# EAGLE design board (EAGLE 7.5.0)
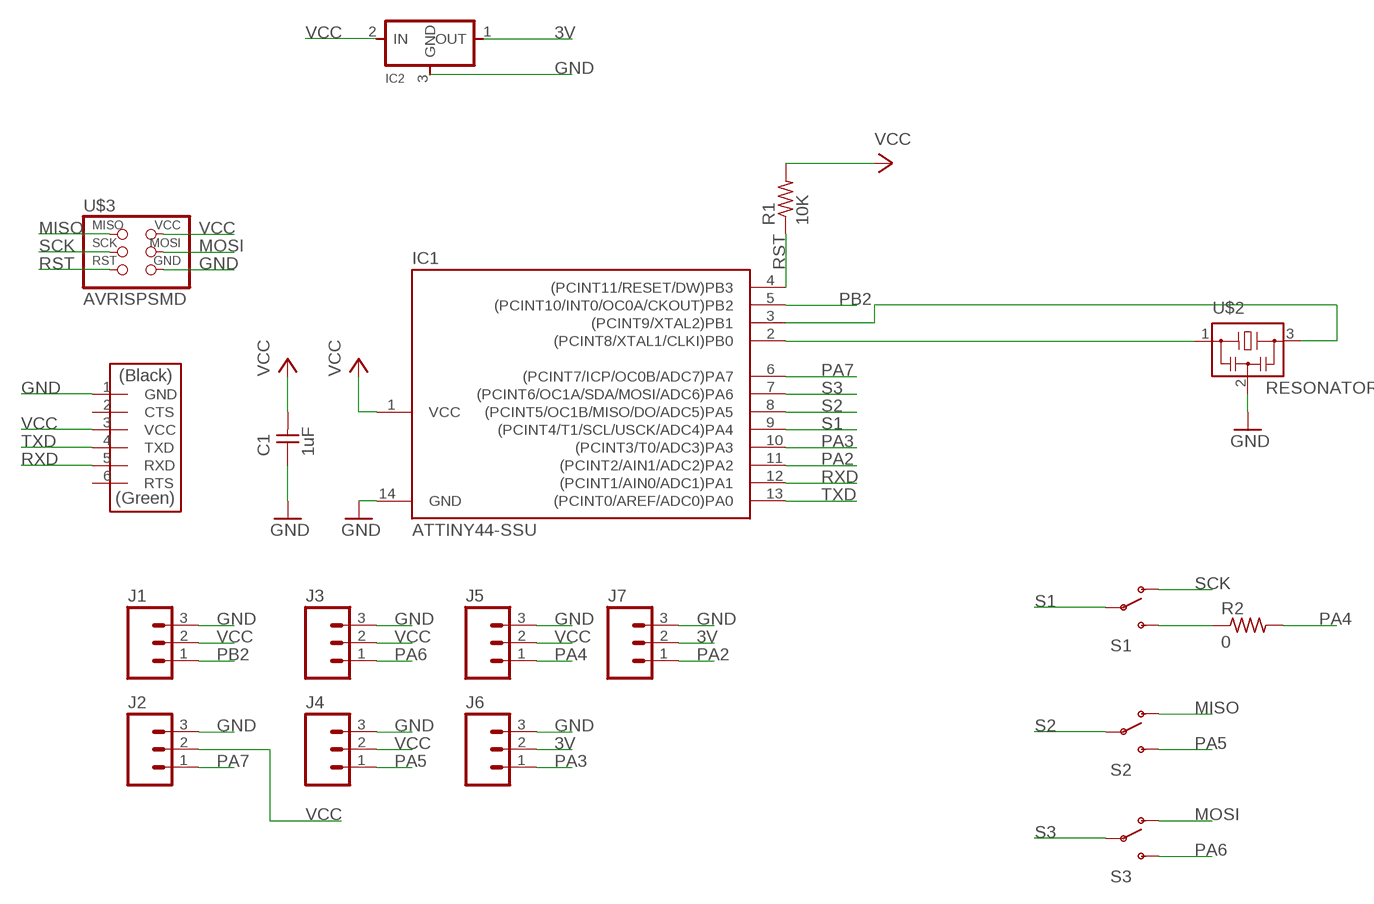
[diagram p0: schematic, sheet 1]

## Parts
C1  1uF  CAP-UNPOLARIZED  [C1206]
IC1  ATTINY44-SSU  [SOIC14]
IC2  REGULATORSOT23  [SOT23]
J1  M03SMD_RA_MALE  [1X03_SMD_RA_MALE]
J2  M03SMD_RA_MALE  [1X03_SMD_RA_MALE]
J3  M03SMD_RA_MALE  [1X03_SMD_RA_MALE]
J4  M03SMD_RA_MALE  [1X03_SMD_RA_MALE]
J5  M03SMD_RA_MALE  [1X03_SMD_RA_MALE]
J6  M03SMD_RA_MALE  [1X03_SMD_RA_MALE]
J7  M03SMD_RA_MALE  [1X03_SMD_RA_MALE]
R1  10K  RES-US1206FAB  [R1206FAB]
R2  0  RES-US1206FAB  [R1206FAB]
S1  SWITCH-SPDTSMD2  [SWITCH-SPDT-SMD]
S2  SWITCH-SPDTSMD2  [SWITCH-SPDT-SMD]
S3  SWITCH-SPDTSMD2  [SWITCH-SPDT-SMD]
U$2  RESONATOR  [EFOBM]
U$3  AVRISPSMD  [2X03SMD]
U$4  FTDI-SMD-HEADER  [1X06SMD]

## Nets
3V: IC2.1(OUT) J6.2 J7.2
GND: C1.1 IC1.14(GND) IC2.3(GND) J1.3 J2.3 J3.3 J4.3 J5.3 J6.3 J7.3 U$2.2 U$3.6(GND) U$4.1(GND)
MISO: S2.1(O) U$3.1(MISO)
MOSI: S3.1(O) U$3.4(MOSI)
N$1: IC1.3((PCINT9/XTAL2)PB1) U$2.3
N$2: IC1.2((PCINT8/XTAL1/CLKI)PB0) U$2.1
N$3: R2.1 S1.3(S)
PA2: IC1.11((PCINT2/AIN1/ADC2)PA2) J7.1
PA3: IC1.10((PCINT3/T0/ADC3)PA3) J6.1
PA4: J5.1 R2.2
PA5: J4.1 S2.3(S)
PA6: J3.1 S3.3(S)
PA7: IC1.6((PCINT7/ICP/OC0B/ADC7)PA7) J2.1
PB2: IC1.5((PCINT10/INT0/OC0A/CKOUT)PB2) J1.1
RST: IC1.4((PCINT11/RESET/DW)PB3) R1.1 U$3.5(RST)
RXD: IC1.12((PCINT1/AIN0/ADC1)PA1) U$4.5(RXD)
S1: IC1.9((PCINT4/T1/SCL/USCK/ADC4)PA4) S1.2(P)
S2: IC1.8((PCINT5/OC1B/MISO/DO/ADC5)PA5) S2.2(P)
S3: IC1.7((PCINT6/OC1A/SDA/MOSI/ADC6)PA6) S3.2(P)
SCK: S1.1(O) U$3.3(SCK)
TXD: IC1.13((PCINT0/AREF/ADC0)PA0) U$4.4(TXD)
VCC: C1.2 IC1.1(VCC) IC2.2(IN) J1.2 J2.2 J3.2 J4.2 J5.2 R1.2 U$3.2(VCC) U$4.3(VCC)
Unconnected: U$4.2(CTS) U$4.6(RTS)

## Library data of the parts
C1 = fab:CAP-UNPOLARIZED
IC1 = fab:ATTINY44
IC2 = fab:REGULATOR
J1-J7 = SparkFun-Connectors:M03: Header 3 Standard 3-pin 0.1" header. Use with straight break away headers (SKU : PRT-00116), right angle break away headers (PRT-00553), swiss pins (PRT-00743), machine pins (PRT-00117), and female headers (PRT-00115). Molex polarized connector foot print use with SKU : PRT-08232 with associated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; PROD_ID: CONN-10925
R1 R2 = fab:RES-US: Resistor (US Symbol)
S1-S3 = SparkFun-Electromechanical:SWITCH-SPDT: SPDT Switch Simple slide switch, Spark Fun Electronics SKU : COM-00102 DPDT SMT slide switch, AYZ0202, SWCH-08179
U$2 = fab:RESONATOR
U$3 = fab:AVRISP
U$4 = fab:FTDI-SMD-HEADER

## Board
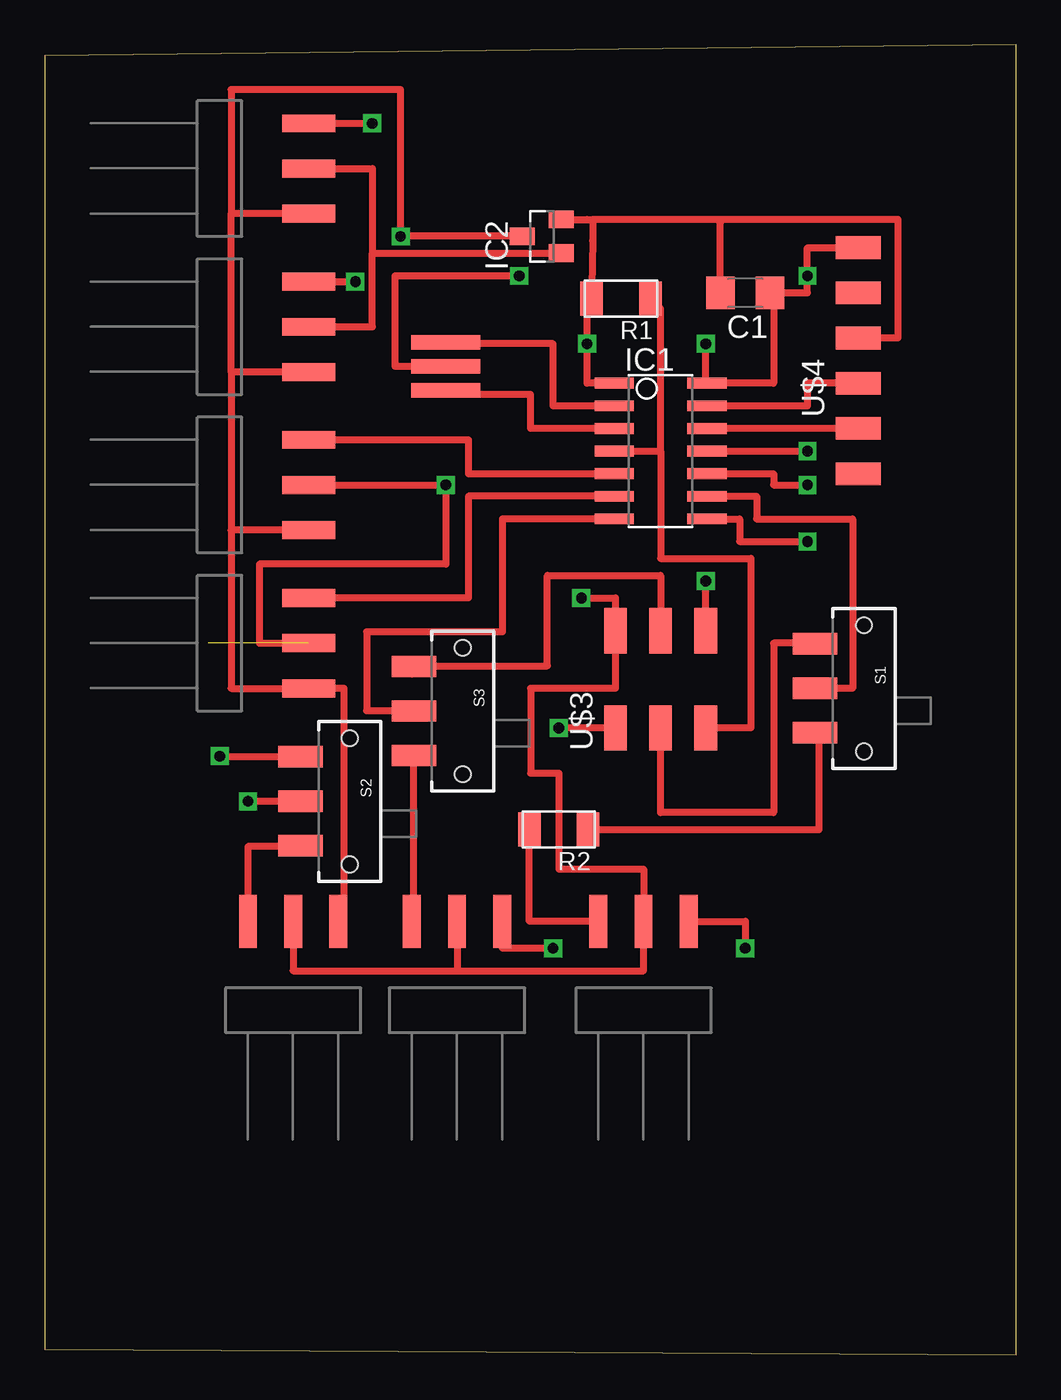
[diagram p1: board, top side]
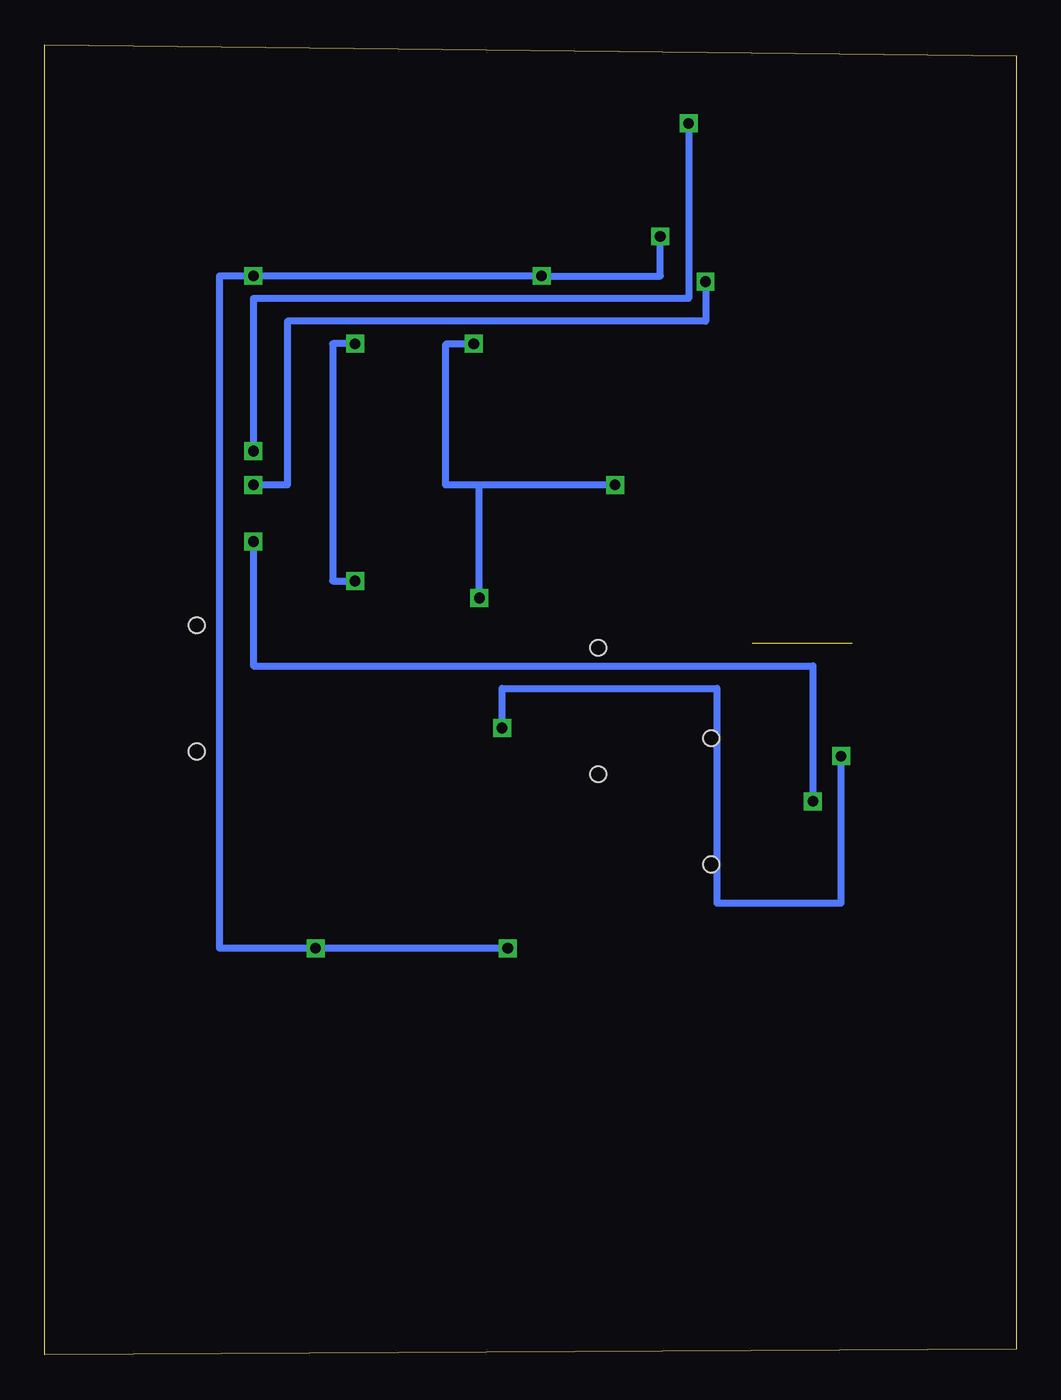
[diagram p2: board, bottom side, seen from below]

Size 54.6 x 73.65 mm. Coordinates in mm from the lower left corner, seen from the top.
Outline: 0,0.32 54.6,0 54.6,73.65 0,73.02 0,0.32
Copper layers (1*16): Top 0.035mm / dielectric 1.5mm / Bottom 0.035mm
Design rules "default": minimum track width 10mil, minimum drill 24mil, track to track 8mil, track to pad 8mil, pad to pad 8mil, via to via 8mil, smd to smd 8mil, copper to edge 40mil, drill to drill 8mil, minimum pad ring 10mil, minimum via ring 8mil, stop-mask expansion 4mil, vias tented up to drill 0mil, thermal gap 10mil

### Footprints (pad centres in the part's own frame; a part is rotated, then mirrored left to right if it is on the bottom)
C1206 = smd 1.6 x 1.8: 1 -1.4,0; 2 1.4,0
SOIC14 = smd 0.61 x 2.21: 1 -3.81,-2.603; 2 -2.54,-2.603; 3 -1.27,-2.603; 4 0,-2.603; 5 1.27,-2.603; 6 2.54,-2.603; 7 3.81,-2.603; 8 3.81,2.603; 9 2.54,2.603; 10 1.27,2.603; 11 0,2.603; 12 -1.27,2.603; 13 -2.54,2.603; 14 -3.81,2.603
SOT23 = smd 1 x 1.4: 1 -0.95,-1.1; 2 0.95,-1.1; 3 0,1.1
1X03_SMD_RA_MALE = smd 1 x 3: 1 -2.54,5; 2 0,5; 3 2.54,5
R1206FAB = smd 1.27 x 1.905: 1 -1.651,0; 2 1.651,0
SWITCH-SPDT-SMD = smd 1.2 x 2.5: 1 -2.5,-2.75; 2 0,-2.75; 3 2.5,-2.75 | hole 0.9: -3.55,0; 3.55,0
EFOBM = smd 0.8 x 3.9: 1 -1.35,0; 2 0,0; 3 1.35,0
2X03SMD = smd 2.54 x 1.27: 1 -2.54,2.54; 2 2.92,2.54; 3 -2.54,0; 4 2.92,0; 5 -2.54,-2.54; 6 2.92,-2.54
1X06SMD = smd 2.54 x 1.27: 1 0,6.35; 2 0,3.81; 3 0,1.27; 4 0,-1.27; 5 0,-3.81; 6 0,-6.35

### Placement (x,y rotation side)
C1  39.37,59.69 180 top
IC1  34.61,50.8 270 top
IC2  27.94,62.87 90 top
J1  9.84,48.9 270 top
J2  9.84,40.01 270 top
J3  23.18,19.37 0 top
J4  13.97,19.37 0 top
J5  33.66,19.37 0 top
J6  9.84,57.79 270 top
J7  9.84,66.67 270 top
R1  32.38,59.37 180 top
R2  28.89,29.53 180 top
S1  46.04,37.47 270 top
S2  17.14,31.11 270 top
S3  23.5,36.2 270 top
U$2  22.54,55.56 270 top
U$3  34.61,37.78 90 top
U$4  45.72,55.88 0 top

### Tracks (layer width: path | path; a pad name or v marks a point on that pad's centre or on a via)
3V
  Top 0.406: 18.41,61.91 25.23,61.91 IC2.1 | J6.2 18.41,57.79 18.41,61.91 | J7.2 18.41,66.68 18.41,61.91
GND  (via drill 0.6)
  Top 0.406: IC2.3 v20,62.86 20,71.12 10.48,71.12 10.48,64.14 | v37.15,56.83 37.15,54.61 IC1.14 40.96,54.61 40.96,59.69 C1.1 42.86,59.69 v42.86,60.64 42.86,62.23 U$4.1 | U$3.6 v37.15,43.5 | J6.3 10.48,55.25 | 10.48,55.25 10.48,64.14 | J7.3 10.48,64.14 | 10.48,55.25 10.48,46.36 | J1.3 10.48,46.36 | 10.48,46.36 10.48,37.47 J2.3 16.83,37.47 16.83,24.68 J4.3 | J5.3 39.37,24.37 v39.37,22.86 | v28.57,22.86 25.72,22.86 J3.3 | v26.67,60.64 19.68,60.64 19.68,55.56 U$2.2
  Bottom 0.406: v37.15,56.83 38.42,56.83 38.42,43.5 v37.15,43.5 | v28.57,22.86 v39.37,22.86 44.77,22.86 44.77,60.64 v42.86,60.64 v26.67,60.64 20,60.64 v20,62.86
MISO  (via drill 0.6)
  Top 0.406: U$3.1 v28.89,35.24 | S2.1 10.16,33.61 v9.84,33.65
  Bottom 0.406: v28.89,35.24 28.89,37.47 16.83,37.47 16.83,25.4 9.84,25.4 v9.84,33.65
MOSI
  Top 0.406: U$3.4 34.61,43.82 28.26,43.82 28.26,38.73 20.64,38.73 20.64,38.27 S3.1
N$1
  Top 0.406: IC1.3 27.3,52.07 27.3,53.97 23.26,53.97 U$2.3
N$2
  Top 0.406: IC1.2 28.57,53.34 28.57,56.83 22.54,56.83 U$2.1
N$3
  Top 0.406: R2.1 43.5,29.53 43.5,34.76 S1.3
PA2  (via drill 0.6)
  Top 0.406: IC1.11 v42.86,50.8 | J7.1 v18.41,69.21
  Bottom 0.406: v18.41,69.21 18.41,59.37 42.86,59.37 v42.86,50.8
PA3  (via drill 0.6)
  Top 0.406: J6.1 v17.46,60.33 | IC1.10 40.96,49.53 40.96,48.9 v42.86,48.9
  Bottom 0.406: v17.46,60.33 17.46,58.1 40.96,58.1 40.96,48.9 v42.86,48.9
PA4
  Top 0.406: J5.1 27.24,24.37 R2.2
PA5
  Top 0.406: S2.3 14.36,28.58 11.43,28.58 J4.1
PA6
  Top 0.406: J3.1 20.64,24.45 20.75,24.56 S3.3
PA7
  Top 0.406: IC1.6 23.81,48.26 23.81,42.54 J2.1
PB2
  Top 0.406: J1.1 23.81,51.43 23.81,49.53 IC1.5
RST
  Top 0.406: IC1.4 34.61,50.8 | 34.61,50.8 34.61,44.77 39.69,44.77 39.69,35.24 U$3.5 | 34.61,50.8 34.61,58.8 R1.1
RXD
  Top 0.406: U$4.5 IC1.12
S1
  Top 0.406: 37.15,48.26 IC1.9 40.01,48.26 40.01,46.99 45.4,46.99 45.4,37.47 S1.2
S2  (via drill 0.6)
  Top 0.406: 37.15,46.99 IC1.8 39.05,46.99 39.05,45.72 v42.86,45.72 | S2.2 v11.43,31.11
  Bottom 0.406: v42.86,45.72 42.86,38.73 11.43,38.73 v11.43,31.11
S3
  Top 0.406: IC1.7 25.72,46.99 25.72,40.64 18.1,40.64 18.1,36.19 S3.2
SCK
  Top 0.406: U$3.3 34.61,30.48 40.96,30.48 40.96,40.01 43.25,40.01 S1.1
TXD
  Top 0.406: U$4.4 42.86,54.61 42.86,53.34 IC1.13
VCC  (via drill 0.6)  (1 unrouted)
  Top 0.406: 30.75,60.01 30.8,62.61 30.8,63.82 | 30.75,60.01 R1.2 | U$4.3 47.94,57.15 47.94,63.82 37.78,63.82 | 32.07,54.61 IC1.1 30.48,54.61 v30.48,56.83 30.48,59.74 30.75,60.01 | IC2.2 30.48,63.82 30.8,63.82 | 14.61,48.9 J1.2 v22.54,48.9 22.54,44.45 12.06,44.45 12.06,40.01 J2.2 | J4.2 13.97,21.59 23.18,21.59 | J3.2 23.18,21.59 | 23.18,21.59 33.66,21.59 J5.2 33.66,27.31 28.89,27.31 28.89,32.7 27.3,32.7 27.3,37.47 32.07,37.47 U$3.2 32.07,42.54 v30.16,42.54 | 37.78,63.82 30.8,63.82 | C1.2 37.97,63.63 37.78,63.82
  Bottom 0.406: v30.48,56.83 32,56.83 32.07,56.77 32.07,48.9 30.16,48.9 | v22.54,48.9 30.16,48.9 | v30.16,42.54 30.16,48.9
